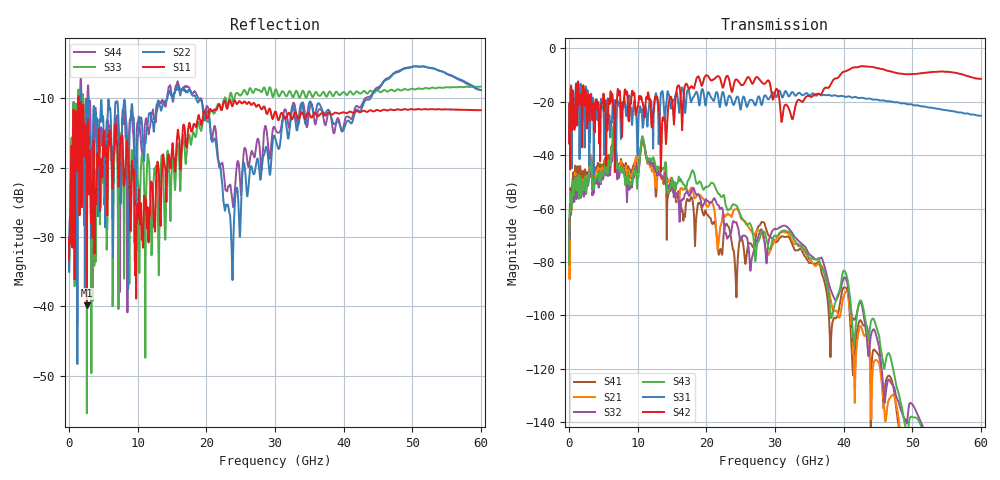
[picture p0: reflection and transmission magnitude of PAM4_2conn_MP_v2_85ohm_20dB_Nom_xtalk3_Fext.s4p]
! Info: Touchstone file created by Circ.  Input file=FAB50GbE_2conn_Midplane_Examax_Topo2_v2_85ohm_20dB_Nom.circ
# Hz S RI R 50
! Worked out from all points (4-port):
!   6000 points, 10 MHz to 60 GHz, reference 50 ohm
!   strongest paths, dB at 10 MHz, 15.01 GHz, 30.01 GHz, 45.01 GHz, 60 GHz:
!     S42: -35.6, -19.6, -16.3, -7.5, -11.4
!     S31: -35.4, -19.8, -17.5, -19.3, -25.2
!     S43: -80.7, -48.6, -70.1, -106.2, -158.1
!     S32: -68.1, -48.7, -67.6, -110.2, -153.1
!     S21: -64.0, -49.5, -72.1, -117.3, -159.3
!     S41: -67.5, -51.5, -72.3, -114.4, -170.3
!   lowest |S11| = -39.8 dB at 2.61 GHz (marker M1), VSWR 1.02, Z = 51 + j0.122 ohm
!   |S11| at or under -10 dB: start of sweep to 1.341 GHz; 1.403 GHz to end of sweep
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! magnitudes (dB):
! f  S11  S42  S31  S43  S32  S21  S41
! 10 MHz  -33.3  -35.6  -35.4  -80.7  -68.1  -64.0  -67.5
! 740 MHz  -15.0  -28.8  -21.0  -55.0  -57.0  -52.8  -49.9
! 2.61 GHz  -39.8  -29.4  -18.5  -48.9  -50.1  -48.3  -47.0
! 10.75 GHz  -31.5  -20.6  -29.7  -33.2  -34.0  -34.5  -33.8
! 21.7 GHz  -11.0  -10.4  -17.7  -54.3  -58.6  -74.8  -75.0
! 24.33 GHz  -10.7  -11.7  -18.9  -58.8  -65.1  -60.2  -89.7
! 60 GHz  -11.7  -11.4  -25.2  -158.1  -153.1  -159.3  -170.3
